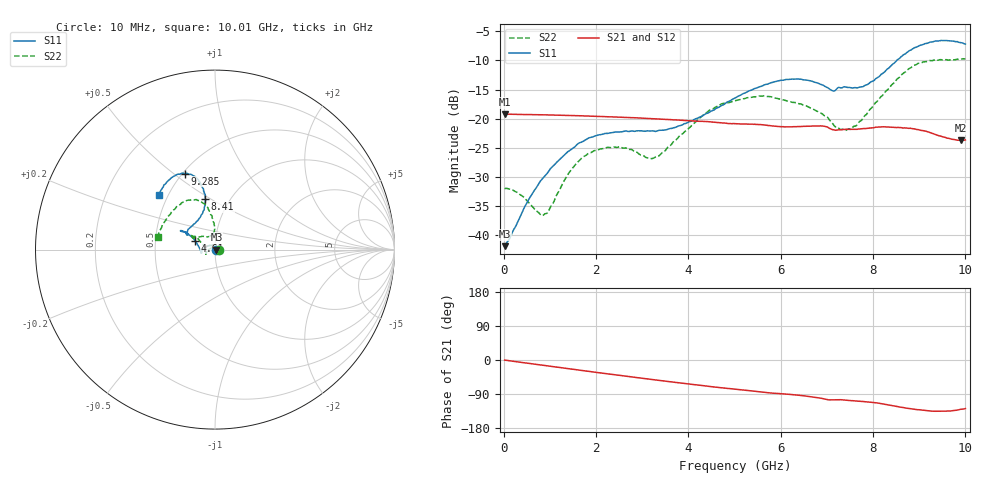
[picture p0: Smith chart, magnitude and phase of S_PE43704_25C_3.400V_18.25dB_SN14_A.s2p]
! Device ID: PE43704
! Dir: z:\PE43704\PE43704_Char_1_20130516\PE43704\AMB\3p400V\18p25dB
! Serial: 14
! Insertion: A
! Impedance: 50 ohm
! Temp: Amb
! VDD: 3.400V
! Attenuation Step: 18.25dB
! IDD: 1.140682e-01mA
#  Hz  S  RI  R  50
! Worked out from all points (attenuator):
!   401 points, 10 MHz to 10.01 GHz, reference 50 ohm
!   highest |S21| = -19.23 dB at 10 MHz (marker M1); lowest = -23.7 dB at 9.91 GHz (marker M2)
!   lowest |S11| = -41.9 dB at 10 MHz (marker M3), VSWR 1.02, Z = 50.8 + j0.0398 ohm
!   |S11| at or under -10 dB: start of sweep to 8.523 GHz
!   |S22| runs from -36.7 to -9.7 dB; largest |S21 - S12| = 0.0011
!   S11 on the Smith chart (normalised r, x): 10 MHz: 1.02, +0.00; 4.61 GHz: 0.79, +0.08; 8.41 GHz: 0.77, +0.48; 9.285 GHz: 0.51, +0.55; 10.01 GHz: 0.45, +0.34
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1e7  0.00802 0.000391  0.1093 -0.000327  0.1093 -0.000368  0.025 0.00024
3.35e8  0.00384 0.0136  0.1082 -0.0108  0.1082 -0.0108  0.0201 0.00985
8.6e8  -0.0194 0.0247  0.1044 -0.0267  0.1044 -0.0266  -0.00266 0.0147
9.85e8  -0.0263 0.0248  0.1032 -0.0302  0.1032 -0.0302  -0.0101 0.0133
1.41e9  -0.0504 0.0159  0.0978 -0.042  0.0978 -0.042  -0.0344 0.000977
1.685e9  -0.0626 0.00672  0.0936 -0.0492  0.0936 -0.0491  -0.045 -0.00963
2.36e9  -0.0746 -0.0139  0.0812 -0.0641  0.0812 -0.0641  -0.0514 -0.0244
3.16e9  -0.0767 -0.0159  0.0635 -0.0776  0.0635 -0.0776  -0.045 -0.00656
3.36e9  -0.0786 -0.0104  0.0586 -0.08  0.0587 -0.08  -0.0478 0.0025
4.61e9  -0.1122 0.0504  0.0286 -0.0882  0.029 -0.0882  -0.1056 0.07
5.01e9  -0.1319 0.0719  0.0208 -0.0881  0.0208 -0.0881  -0.1221 0.0735
5.96e9  -0.1831 0.1051  0.00219 -0.0854  0.00236 -0.0855  -0.1281 0.0736
6.685e9  -0.1838 0.1003  -0.0109 -0.0855  -0.0109 -0.0856  -0.1015 0.0675
7.135e9  -0.1506 0.0852  -0.021 -0.0774  -0.0211 -0.0776  -0.055 0.0713
7.485e9  -0.1364 0.1255  -0.0234 -0.0774  -0.0233 -0.0777  -0.0223 0.0784
7.835e9  -0.0906 0.1705  -0.0284 -0.077  -0.0281 -0.0769  -0.00374 0.1069
8.36e9  -0.0534 0.2696  -0.0409 -0.0743  -0.0408 -0.0743  -0.0162 0.1837
8.41e9  -0.054 0.2833  -0.0423 -0.0729  -0.042 -0.0733  -0.0224 0.1936
8.86e9  -0.0917 0.3855  -0.0521 -0.0635  -0.0513 -0.0636  -0.0802 0.2692
9.285e9  -0.1664 0.4236  -0.0529 -0.0529  -0.0532 -0.0531  -0.1658 0.2674
9.91e9  -0.2958 0.3375  -0.0419 -0.0499  -0.0422 -0.0493  -0.3036 0.1124
1.001e10  -0.3125 0.3056  -0.0405 -0.0516  -0.0415 -0.0517  -0.3188 0.0713
